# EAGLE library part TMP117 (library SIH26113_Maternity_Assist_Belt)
TI TMP117AIDRVR high-accuracy digital temperature sensor, WSON-6 (DRV). +/-0.1 C, 1.8-5.5 V, I2C. Pin map from TMP117 SNOSD82D Table 5-1 (WSON column).
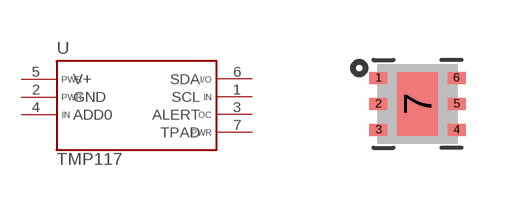
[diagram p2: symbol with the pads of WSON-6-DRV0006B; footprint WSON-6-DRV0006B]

Designator prefix U

## TMP117  [WSON-6-DRV0006B]
1  SCL  in
2  GND  pwr
3  ALERT  oc
4  ADD0  in
5  V+  pwr
6  SDA
7  TPAD  pwr

## Footprint WSON-6-DRV0006B (pad centres in mm)
TI DRV0006B 6-pin WSON 2.0x2.0 mm, 0.65 mm pitch, thermal pad 1.0x1.6 mm. Lands 0.45x0.30 mm at 1.95 mm row spacing, taken directly from TI's EXAMPLE BOARD LAYOUT (TMP117 SNOSD82D p.41). Pad 7 =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
smd 0.45 x 0.3: 1 -0.975,0.65; 2 -0.975,0; 3 -0.975,-0.65; 4 0.975,-0.65; 5 0.975,0; 6 0.975,0.65
smd 1 x 1.6: 7 0,0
